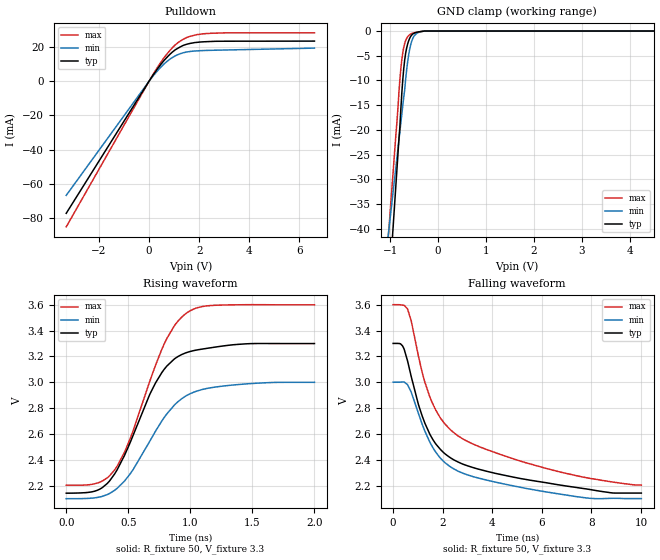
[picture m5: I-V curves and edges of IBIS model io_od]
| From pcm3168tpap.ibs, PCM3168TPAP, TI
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[Model]   io_od
Model_type I/O_open_drain
Vinl=8.000E-01
Vinh=2.000E+00
Vref=3.300E+00
Rref=1.000E+06
Cref=0.000E+00
Vmeas=1.650E+00
C_comp   880.000fF   880.000fF   880.000fF
[Voltage Range]   3.300E+00   3.000E+00   3.600E+00
[POWER Clamp Reference]   3.300E+00   3.000E+00   3.600E+00
[GND Clamp Reference]   0.000E+00   0.000E+00   0.000E+00
[Pullup Reference]   3.300E+00   3.000E+00   3.600E+00
[Pulldown Reference]   0.000E+00   0.000E+00   0.000E+00
[Temperature Range]   25   105   -40
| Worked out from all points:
|   slope of the pulldown table from 0 to 0.495 V, typ, clamps not added: 47.9 ohm
|   GND clamp passes 1 mA (typ) near -0.57 V on its own axis
|   rising waveform, R_fixture 50, V_fixture 3.3: 20-80 % time 329ps typ, 362ps min, 321ps max; typ from 2.14 V to 3.3 V
|   falling waveform, R_fixture 50, V_fixture 3.3: 20-80 % time 2.02ns typ, 2.14ns min, 2.82ns max; typ from 3.3 V to 2.14 V
[GND Clamp]
-3.3V     -385.7mA   -236.3mA   -336.8mA
-880mV    -30.73mA   -27.26mA   -20.59mA
-800mV    -19.42mA   -20.35mA   -9.852mA
-780mV    -15.87mA   -18.62mA   -7.632mA
-740mV    -9.961mA   -15.16mA   -4.443mA
-720mV    -7.709mA   -13.43mA   -3.354mA
-660mV    -3.514mA   -7.992mA   -1.511mA
-620mV    -2.074mA   -5.051mA   -956.6uA
-560mV    -886.6uA   -2.284mA   -532.8uA
-440mV    -233.2uA   -396.9uA   -223.7uA
-280mV    0A         0A         0A
6.6V      0A         0A         0A
[Pulldown]
-3.3V     -77.4mA    -66.86mA   -85.34mA
140mV     3.167mA    2.696mA    3.525mA
620mV     12.54mA    10.43mA    14.23mA
920mV     17.01mA    13.85mA    19.51mA
1.1V      18.97mA    15.3mA     22.02mA
1.5V      21.72mA    17.19mA    25.66mA
1.9V      22.83mA    17.86mA    27.34mA
2.2V      23.2mA     18.08mA    27.92mA
3.06V     23.53mA    18.38mA    28.44mA
6.6V      23.6mA     19.49mA    28.45mA
[Rising Waveform]
R_fixture = 50
V_fixture = 3.3
V_fixture_min = 3
V_fixture_max = 3.6
0s        2.142V     2.099V     2.204V
250ps     2.164V     2.109V     2.22V
390ps     2.291V     2.164V     2.322V
510ps     2.522V     2.285V     2.552V
720ps     2.996V     2.623V     3.133V
790ps     3.102V     2.729V     3.298V
870ps     3.18V      2.823V     3.436V
970ps     3.23V      2.898V     3.537V
1.18ns    3.27V      2.96V      3.595V
2ns       3.3V       3V         3.6V
[Falling Waveform]
R_fixture = 50
V_fixture = 3.3
V_fixture_min = 3
V_fixture_max = 3.6
0s        3.3V       3V         3.6V
380ps     3.281V     3.002V     3.597V
580ps     3.167V     2.981V     3.568V
730ps     3.044V     2.923V     3.476V
1.02ns    2.828V     2.759V     3.202V
1.5ns     2.591V     2.529V     2.877V
1.95ns    2.471V     2.403V     2.712V
2.6ns     2.384V     2.313V     2.587V
6.22ns    2.221V     2.15V      2.33V
10.01ns   2.142V     2.099V     2.204V
[Ramp]
dV/dt_f   6.9475E-01/2.0186E-09   5.4036E-01/2.1319E-09   8.3763E-01/2.8125E-09
dV/dt_r   6.9475E-01/3.2660E-10   5.4036E-01/3.6170E-10   8.3763E-01/3.2070E-10
R_load = 50
